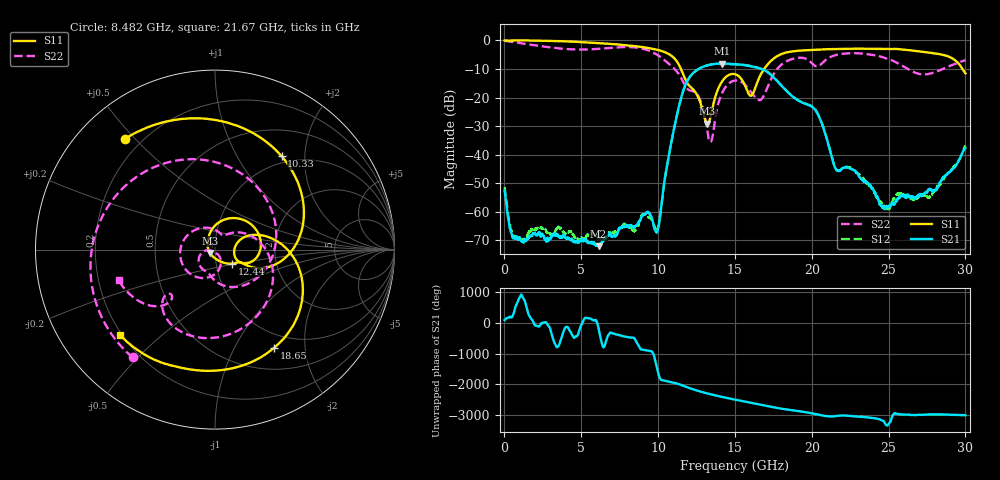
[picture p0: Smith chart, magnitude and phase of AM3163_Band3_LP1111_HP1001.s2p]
!Agilent Technologies,E8364B,MY43040894,A.07.50.67
!Agilent E8364B: A.07.50.67
!Date: Thursday, August 20, 2020 12:17:54
!Correction: S11(Full 2 Port(1,2))
!S21(Full 2 Port(1,2))
!S12(Full 2 Port(1,2))
!S22(Full 2 Port(1,2))
!S2P File: Measurements: S11, S21, S12, S22:
# Hz S  dB  R 50
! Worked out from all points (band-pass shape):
!   3201 points, 10 MHz to 30 GHz, reference 50 ohm
!   highest |S21| = -8.08 dB at 14.15 GHz (marker M1); lowest = -72.1 dB at 6.13 GHz (marker M2)
!   |S21| within 3 dB of the highest: 12.35 GHz to 17.12 GHz (4.772 GHz wide, 32.4 % of centre)
!   lowest |S11| = -29.1 dB at 13.21 GHz (marker M3), VSWR 1.07, Z = 47.1 - j1.72 ohm
!   |S11| at or under -10 dB: 11.49 GHz to 16.9 GHz (5.414 GHz wide, 38.1 % of centre); 29.8 GHz to end of sweep
!   |S22| runs from -35.6 to -0.1 dB; largest |S21 - S12| = 0.012
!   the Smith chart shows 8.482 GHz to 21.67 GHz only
!   S11 on the Smith chart (normalised r, x): 8.482 GHz: 0.14, +0.47; 10.33 GHz: 0.89, +1.56; 12.44 GHz: 1.19, -0.19; 18.65 GHz: 0.80, -1.47; 21.67 GHz: 0.19, -0.37
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1e7  -0.03 -1.9  -52.65 87.0  -51.44 -45.4  -0.13 -5.1
5.160812e8  -0.01 -13.9  -68.84 -150.3  -67.75 -37.5  -0.52 -36.0
1.247088e9  -0.00 -33.8  -70.23 56.3  -69.56 -17.7  -1.12 -82.3
2.662241e9  -0.10 -72.0  -69.68 18.5  -66.49 66.1  -2.22 -162.9
5.014581e9  -0.57 -133.5  -70.09 -65.3  -69.24 -161.9  -3.20 73.2
6.129834e9  -0.92 -162.9  -72.08 160.9  -68.72 90.9  -2.93 11.6
7.516872e9  -1.48 158.8  -65.69 -49.5  -65.79 -53.5  -2.34 -68.1
8.482175e9  -1.99 128.9  -65.39 -169.9  -66.50 -141.9  -2.43 -127.4
1.000979e10  -3.37 70.0  -65.78 160.4  -65.53 -172.4  -5.27 115.4
1.032843e10  -3.89 54.4  -52.55 -74.5  -52.90 -71.5  -6.51 82.9
1.146243e10  -9.71 -16.4  -20.83 145.0  -20.94 145.3  -12.79 -65.3
1.243711e10  -18.20 -39.4  -10.69 -28.3  -10.74 -27.7  -18.28 -134.7
1.32056e10  -29.15 -148.4  -8.72 -136.2  -8.70 -136.1  -31.94 -168.7
1.415216e10  -14.45 66.3  -8.08 111.9  -8.23 111.8  -18.56 -81.3
1.5005e10  -11.82 4.5  -8.29 23.6  -8.39 25.1  -14.05 -150.8
1.664508e10  -12.32 19.9  -9.82 -137.5  -9.80 -136.9  -20.89 59.9
1.865066e10  -3.90 -58.7  -19.17 43.7  -19.11 44.2  -6.64 -72.4
2.000958e10  -3.35 -98.9  -23.21 -60.3  -23.01 -59.7  -8.00 -136.4
2.16684e10  -2.96 -138.1  -45.61 -142.9  -45.45 -142.6  -4.98 -162.5
2.500479e10  -3.01 145.0  -58.41 -41.7  -58.95 -151.1  -6.55 68.3
2.740399e10  -4.09 78.1  -53.49 -105.7  -55.02 -114.3  -11.90 -88.3
3e10  -11.54 -27.6  -37.74 -125.0  -36.80 -125.5  -6.94 131.0
